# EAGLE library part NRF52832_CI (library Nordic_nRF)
nRF52832 Features Single chip, highly flexible, 2.4 GHz multi-protocol SoC 32-bit ARM Cortex-M4F Processor 1.7v to 3.6v operation 512kB flash + 64kB RAM Supports concurrent Bluetooth Smart/ANT protocol operation On-chip NFC tag for Out-of-Band (OOB) pairing Up to +4dBm output power -96dBm sensitivity, Bluetooth Smart Thread safe and run-time protected Event driven API On air compatible with nRF24L and nRF24AP series 2 data rates (2Mbps/1Mbps) PPI - maximum flexibility for power-efficient applications and code simplification Automated power management system with automatic power management of each peripheral Configurable I/O mapping for analog and digital I/O 3 x Master/Slave SPI 2 x Two-wire interface (I²C) UART (RTS/CTS) 3 x PWM AES HW encryption Real Time Counter (RTC) Digital microphone interface (PDM) On-chip balun Applications Internet of Things (IoT) Wearables SmartHome sensors Connected white goods Computer peripherals Voice-command smart remotes A4WP ‘Rezence’ wireless charging Beacons Sports and fitness sensors and hubs Connected health products Smart watches RC Toys Interactive games Building automation and sensor networks
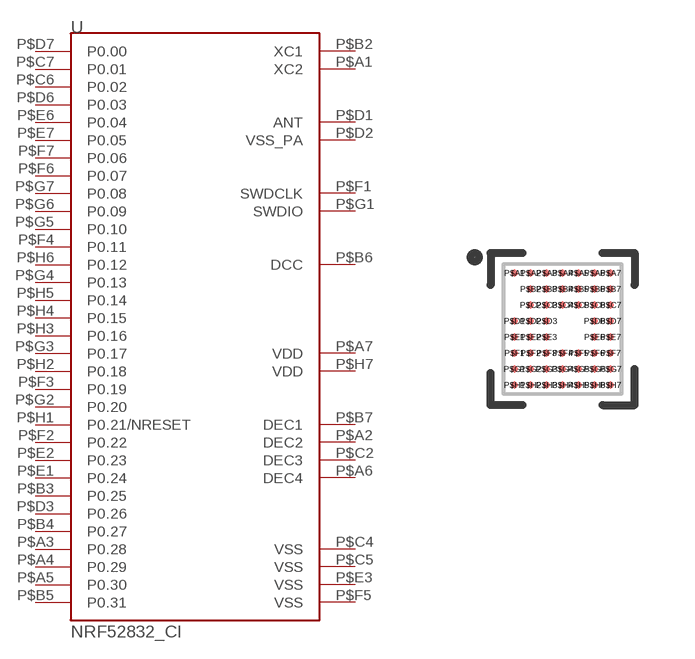
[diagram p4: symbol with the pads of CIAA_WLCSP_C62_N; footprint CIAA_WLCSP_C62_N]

Designator prefix -

## NRF52832_CI  [CIAA_WLCSP_C62_N]
P$A1  XC2
P$A2  DEC2  pwr
P$A3  P0.28
P$A4  P0.29
P$A5  P0.30
P$A6  DEC4  pwr
P$A7  VDD  pwr
P$B2  XC1
P$B3  P0.25
P$B4  P0.27
P$B5  P0.31
P$B6  DCC  pwr
P$B7  DEC1  pwr
P$C2  DEC3  pwr
P$C4  VSS  pwr
P$C5  VSS  pwr
P$C6  P0.02
P$C7  P0.01
P$D1  ANT
P$D2  VSS_PA
P$D3  P0.26
P$D6  P0.03
P$D7  P0.00
P$E1  P0.24
P$E2  P0.23
P$E3  VSS  pwr
P$E6  P0.04
P$E7  P0.05
P$F1  SWDCLK  in
P$F2  P0.22
P$F3  P0.19
P$F4  P0.11
P$F5  VSS  pwr
P$F6  P0.07
P$F7  P0.06
P$G1  SWDIO
P$G2  P0.20
P$G3  P0.17
P$G4  P0.13
P$G5  P0.10
P$G6  P0.09
P$G7  P0.08
P$H1  P0.21/NRESET
P$H2  P0.18
P$H3  P0.16
P$H4  P0.15
P$H5  P0.14
P$H6  P0.12
P$H7  VDD  pwr

## Footprint CIAA_WLCSP_C62_N (pad centres in mm)
CIAA WLCSP package
smd 0.18 x 0.18: P$A1 -1.2,1.4; P$A2 -0.8,1.4; P$A3 -0.4,1.4; P$A4 0,1.4; P$A5 0.4,1.4; P$A6 0.8,1.4; P$A7 1.2,1.4; P$B2 -0.8,1; P$B3 -0.4,1; P$B4 0,1; P$B5 0.4,1; P$B6 0.8,1; P$B7 1.2,1; P$C2 -0.8,0.6; P$C3 -0.4,0.6; P$C4 0,0.6; P$C5 0.4,0.6; P$C6 0.8,0.6; P$C7 1.2,0.6; P$D1 -1.2,0.2; P$D2 -0.8,0.2; P$D3 -0.4,0.2; P$D6 0.8,0.2; P$D7 1.2,0.2; P$E1 -1.2,-0.2; P$E2 -0.8,-0.2; P$E3 -0.4,-0.2; P$E6 0.8,-0.2; P$E7 1.2,-0.2; P$F1 -1.2,-0.6; P$F2 -0.8,-0.6; P$F3 -0.4,-0.6; P$F4 0,-0.6; P$F5 0.4,-0.6; P$F6 0.8,-0.6; P$F7 1.2,-0.6; P$G1 -1.2,-1; P$G2 -0.8,-1; P$G3 -0.4,-1; P$G4 0,-1; P$G5 0.4,-1; P$G6 0.8,-1; P$G7 1.2,-1; P$H1 -1.2,-1.4; P$H2 -0.8,-1.4; P$H3 -0.4,-1.4; P$H4 0,-1.4; P$H5 0.4,-1.4; P$H6 0.8,-1.4; P$H7 1.2,-1.4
